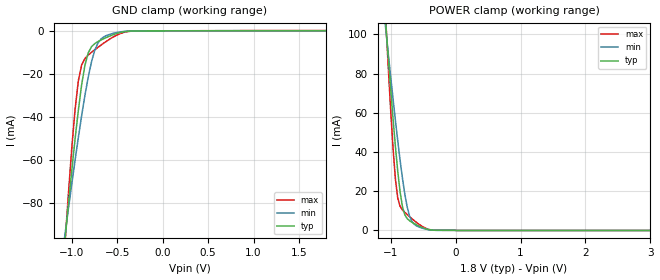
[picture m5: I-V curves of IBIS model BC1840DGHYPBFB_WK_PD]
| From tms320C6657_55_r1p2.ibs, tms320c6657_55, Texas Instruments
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|   Model Cell BC1840DGHYPBFB_WK_PD_ON_1P8
|BC1840DGHYPBFB_WK_PD_ON_1P8
[Model]   BC1840DGHYPBFB_WK_PD
Model_type   Input
Polarity   Non-Inverting
Vinl =  0.63
Vinh =  1.17
C_comp   1.10911p   1.03952p   1.18892p
[Model Spec]
Vinl   0.63   0.5985   0.6615
Vinh   1.17   1.1115   1.2285
D_overshoot_high 2.34 2.34 2.34
D_overshoot_low -0.3 -0.3 -0.3
D_overshoot_time 1.00E-09 1.00E-09 1.00E-09
S_overshoot_high 1.98 1.98 1.98
S_overshoot_low 0 0 0
[Temperature Range]   25   105   -40
[Voltage Range]   1.8   1.71   1.89
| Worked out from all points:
|   GND clamp passes 1 mA (typ) near -0.49 V on its own axis
|   POWER clamp passes 1 mA (typ) near -0.47 V on its own axis
[POWER_clamp]
|   voltage   I(typ)   I(min)   I(max)
-1.8V     457.5mA    350.7mA    618.6mA
-1.073V   104mA      101.6mA    105.5mA
-963.6mV  57.09mA    67.13mA    41.97mA
-927.3mV  42.91mA    56.2mA     26.33mA
-890.9mV  30.12mA    45.68mA    16.51mA
-854.5mV  19.54mA    35.72mA    12.28mA
-818.2mV  12.06mA    26.54mA    10.44mA
-745.5mV  6.045mA    11.94mA    8.096mA
-672.7mV  4.189mA    4.584mA    6mA
-600mV    2.844mA    2.294mA    4.061mA
-309.1mV  110.9uA    91.59uA    146.8uA
3.6V      0A         0A         0A
[GND_clamp]
|   voltage   I(typ)   I(min)   I(max)
-1.8V     -448.8mA   -342.6mA   -610mA
-1.073V   -96.81mA   -94.35mA   -98.22mA
-1.036V   -80.81mA   -82.79mA   -75.84mA
-963.6mV  -50.62mA   -60.41mA   -36.84mA
-927.3mV  -37.02mA   -49.73mA   -23.29mA
-890.9mV  -25.16mA   -39.53mA   -15.92mA
-854.5mV  -16.01mA   -30.03mA   -12.9mA
-818.2mV  -10.24mA   -21.48mA   -11.28mA
-745.5mV  -5.911mA   -8.917mA   -8.775mA
-636.4mV  -3.426mA   -2.542mA   -5.368mA
-345.5mV  -94.3uA    -70uA      -148.7uA
1.8V      87.08uA    51.66uA    129.7uA
